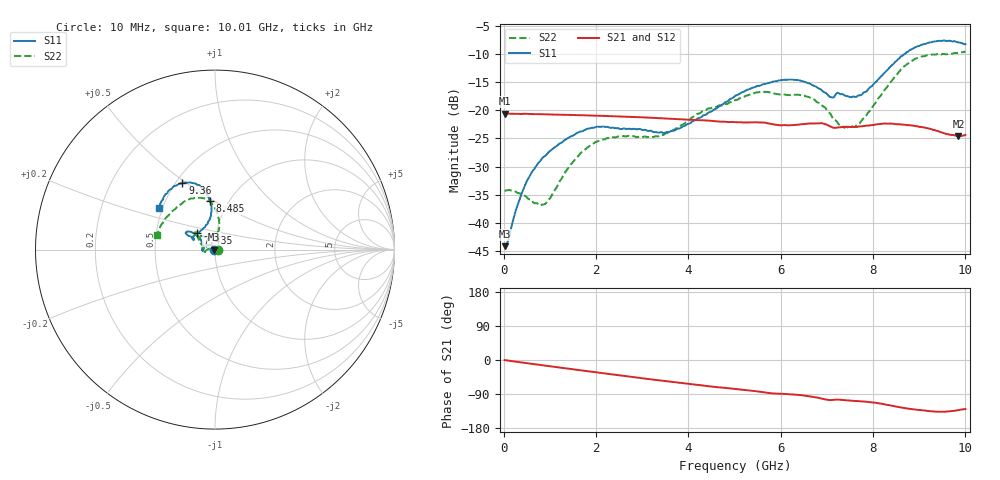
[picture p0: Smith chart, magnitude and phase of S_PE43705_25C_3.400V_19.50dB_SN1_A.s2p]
! Device ID: PE43705
! Serial: 1
! Insertion: A
! Impedance: 50 ohm
! Temp: 25C
! VDD: 3.400V
! Attenuation Step: 19.50dB
#  Hz  S  RI  R  50
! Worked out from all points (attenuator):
!   401 points, 10 MHz to 10.01 GHz, reference 50 ohm
!   highest |S21| = -20.56 dB at 10 MHz (marker M1); lowest = -24.6 dB at 9.86 GHz (marker M2)
!   lowest |S11| = -44.2 dB at 10 MHz (marker M3), VSWR 1.01, Z = 49.4 + j0.0466 ohm
!   |S11| at or under -10 dB: start of sweep to 8.678 GHz
!   |S22| runs from -37.0 to -9.5 dB; largest |S21 - S12| = 0.001
!   S11 on the Smith chart (normalised r, x): 10 MHz: 0.99, +0.00; 7.435 GHz: 0.81, +0.15; 8.485 GHz: 0.82, +0.48; 9.36 GHz: 0.54, +0.48; 10.01 GHz: 0.48, +0.26
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1e7  -0.00615 0.000472  0.0938 -0.000404  0.0939 -0.000368  0.0192 0.000248
8.5e7  -0.0059 0.0035  0.0935 -0.00248  0.0935 -0.00245  0.0194 0.00195
4.6e8  -0.0117 0.0184  0.0923 -0.0127  0.0923 -0.0125  0.0129 0.0114
8.6e8  -0.0285 0.0261  0.0896 -0.0229  0.0896 -0.0228  -0.00373 0.014
1.685e9  -0.0632 0.0157  0.0804 -0.0419  0.0803 -0.0418  -0.0425 0.000277
2.26e9  -0.0708 -0.000992  0.0715 -0.0533  0.0716 -0.0531  -0.0555 -0.012
3.36e9  -0.0633 0.00202  0.0504 -0.0688  0.0506 -0.0686  -0.059 0.00247
3.86e9  -0.0669 0.0247  0.0404 -0.0728  0.0404 -0.0727  -0.0707 0.0228
4.385e9  -0.0769 0.0506  0.0299 -0.0756  0.0301 -0.0754  -0.0875 0.0507
5.01e9  -0.1042 0.0847  0.0185 -0.0765  0.0186 -0.0765  -0.0985 0.0744
5.535e9  -0.1341 0.0976  0.00868 -0.0776  0.00877 -0.0776  -0.1118 0.0926
6.01e9  -0.1575 0.0987  0.00134 -0.0737  0.00147 -0.0737  -0.1053 0.0908
6.685e9  -0.1492 0.0786  -0.00955 -0.076  -0.00951 -0.0759  -0.0979 0.0795
7.085e9  -0.116 0.0615  -0.0194 -0.0694  -0.0194 -0.0691  -0.0575 0.0729
7.435e9  -0.0976 0.0923  -0.0204 -0.0684  -0.0201 -0.0685  -0.0196 0.0689
7.76e9  -0.0547 0.1274  -0.0239 -0.0679  -0.0234 -0.0684  0.00761 0.0811
8.36e9  -0.0195 0.2397  -0.0375 -0.0666  -0.0375 -0.0667  0.0201 0.1725
8.485e9  -0.0263 0.2692  -0.0407 -0.0638  -0.0405 -0.0643  0.0123 0.2012
8.885e9  -0.0788 0.3487  -0.0475 -0.0557  -0.0465 -0.056  -0.0458 0.2784
9.36e9  -0.1819 0.3699  -0.048 -0.0461  -0.0478 -0.0461  -0.1552 0.2739
9.86e9  -0.2892 0.2786  -0.0398 -0.0437  -0.0401 -0.0437  -0.2908 0.1488
1.001e10  -0.3141 0.2309  -0.0384 -0.0468  -0.0386 -0.0468  -0.3259 0.0838
